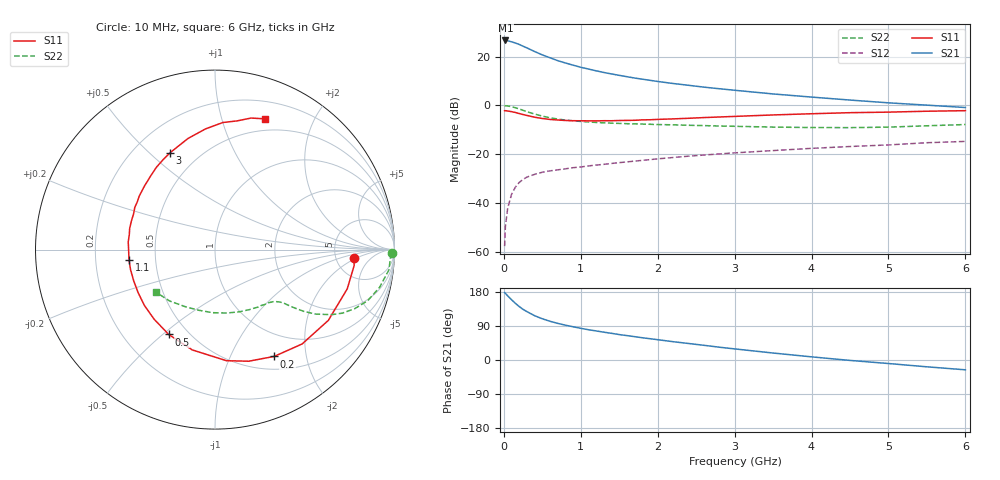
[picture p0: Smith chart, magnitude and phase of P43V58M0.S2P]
! SIEMENS Small Signal Semiconductors
! BFP182
! Si NPN RF Bipolar Junction Transistor in SOT143
! VCE = 3.5 V  IC = 8 mA
! Common Emitter S-Parameters:  March  1996
# GHz  S  MA  R  50
!  f  S11  S21  S12  S22
! GHz  MAG  ANG  MAG  ANG  MAG  ANG  MAG  ANG
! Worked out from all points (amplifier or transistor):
!   36 points, 10 MHz to 6 GHz, reference 50 ohm
!   highest |S21| = 26.6 dB at 20 MHz (marker M1)
!   |S21| within 3 dB of that: start of sweep to 295.9 MHz
!   unconditionally stable (mu >= 1): 1.306 GHz to 5.398 GHz
!   at 250 MHz: K = 0.28, MSG = 27.3 dB, |S12| = -30.3 dB
!   at 1.4 GHz: K = 1.03, MAG = 17.2 dB, |S12| = -23.8 dB
!   at 6 GHz: K = 0.94, MSG = 6.9 dB, |S12| = -14.8 dB
!   lowest NFmin = 1.40 dB at 450 MHz
!   S11 on the Smith chart (normalised r, x): 10 MHz: 7.53, -1.69; 200 MHz: 0.67, -1.48; 500 MHz: 0.39, -0.52; 1.1 GHz: 0.35, -0.05; 3 GHz: 0.35, +0.58; 6 GHz: 0.37, +1.38
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0.01  0.7756 -3.3  21.28 177.8  0.0013 81.9  0.9852 -1.2
0.02  0.7802 -6.6  21.46 175.9  0.0033 82.8  0.9788 -2.7
0.05  0.7686 -16.5  21.11 169.3  0.0078 84.6  0.9752 -6.7
0.1  0.7444 -32.0  20.14 159.1  0.015 73.0  0.9403 -13.0
0.15  0.7155 -47.3  19.02 149.5  0.0211 66.6  0.8972 -18.5
0.2  0.6804 -61.0  17.78 141.0  0.0263 61.9  0.8453 -22.9
0.25  0.6496 -73.2  16.35 133.6  0.0304 57.1  0.7933 -26.5
0.3  0.6224 -84.1  15.09 127.7  0.0339 53.7  0.7433 -29.2
0.4  0.5731 -102.8  12.73 116.9  0.0386 48.5  0.6646 -32.7
0.5  0.5386 -118.6  10.85 108.8  0.0426 44.3  0.6034 -34.8
0.6  0.5153 -131.1  9.48 102.2  0.0455 43.4  0.5584 -36.0
0.7  0.5017 -141.5  8.278 96.7  0.0477 41.9  0.5255 -36.9
0.9  0.4855 -158.6  6.685 87.7  0.0529 41.1  0.4831 -38.0
1.1  0.4826 -173.4  5.568 79.9  0.0575 41.3  0.4574 -39.5
1.3  0.4853 175.0  4.733 73.4  0.0619 41.2  0.4393 -41.2
1.6  0.4926 160.5  3.878 64.4  0.0694 41.4  0.4218 -44.5
2.2  0.5289 138.0  2.814 48.3  0.0855 40.3  0.3999 -53.2
3  0.5949 114.9  2.044 29.3  0.1064 36.4  0.3727 -68.4
3.5  0.6374 103.6  1.718 18.4  0.1186 33.2  0.3593 -79.6
4.5  0.7093 86.5  1.287 -1.1  0.1436 26.7  0.35 -105.2
5.5  0.7599 74.7  1.012 -18.0  0.1717 19.9  0.3821 -131.5
6  0.7794 69.2  0.905 -25.9  0.1827 15.4  0.4054 -144.1
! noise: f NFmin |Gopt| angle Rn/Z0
0.45  1.4  0.26  41  0.29
0.9  1.5  0.25  83  0.23
1.8  2  0.21  162  0.2
